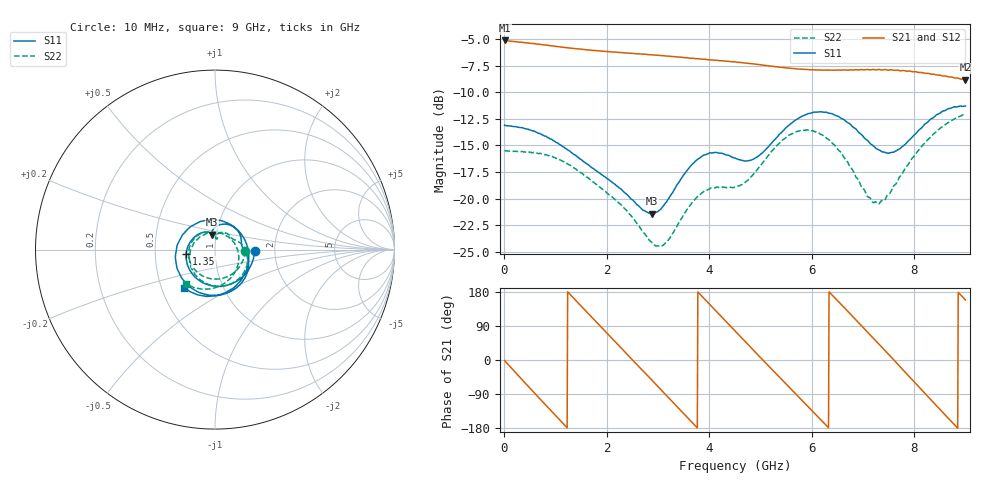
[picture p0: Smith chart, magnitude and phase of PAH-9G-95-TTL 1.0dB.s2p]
! MTS Systemtechnik GmbH
! S-Parameters
! Model: PAH-9G/95-TTL
! Attenuation Step: 1.0dB
#  HZ  S  DB  R  50.00
! Rohde & Schwarz Vector Network Analyzer
! Rohde-Schwarz,ZNB20-2Port,1334333062101652,3.45
! Created: UTC 1/26/2024, 7:17:38 AM
! freq[Hz]  db:S11  ang:S11  db:S21  ang:S21  db:S12  ang:S12  db:S22  ang:S22
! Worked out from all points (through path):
!   900 points, 10 MHz to 9 GHz, reference 50 ohm
!   highest |S21| = -5.13 dB at 10 MHz (marker M1); lowest = -8.8 dB at 9 GHz (marker M2)
!   group delay of S21, straight-line fit = 393 ps
!   lowest |S11| = -21.4 dB at 2.88 GHz (marker M3), VSWR 1.19, Z = 47.8 + j8.02 ohm
!   |S11| at or under -10 dB: start of sweep to end of sweep
!   |S22| runs from -24.5 to -12.1 dB; largest |S21 - S12| = 0.015
!   S11 on the Smith chart (normalised r, x): 10 MHz: 1.57, -0.03; 1.35 GHz: 0.72, -0.04; 9 GHz: 0.65, -0.30
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1e7  -13.10 -2.3  -5.13 -1.5  -5.13 -1.5  -15.47 -2.8
6.4e8  -13.78 -88.6  -5.47 -94.0  -5.47 -93.9  -15.72 -100.6
1.02e9  -14.73 -136.3  -5.69 -148.8  -5.70 -148.7  -16.23 -153.0
1.35e9  -15.81 -171.5  -5.88 164.1  -5.88 164.3  -17.07 169.0
1.51e9  -16.34 173.7  -5.96 141.3  -5.97 141.5  -17.59 152.8
1.91e9  -17.77 141.6  -6.13 84.7  -6.14 84.8  -19.10 120.1
2.32e9  -19.30 115.3  -6.28 26.6  -6.29 26.6  -20.80 94.1
2.88e9  -21.42 100.8  -6.48 -52.7  -6.48 -52.8  -24.11 78.3
3.01e9  -21.18 101.5  -6.53 -71.3  -6.53 -71.2  -24.47 81.2
3.34e9  -19.00 95.2  -6.65 -118.4  -6.66 -117.7  -22.88 86.9
3.76e9  -16.37 69.5  -6.84 -177.7  -6.85 -177.3  -19.88 70.0
4.17e9  -15.70 39.0  -7.00 124.3  -7.01 124.7  -18.93 46.5
4.51e9  -16.21 18.3  -7.15 76.2  -7.15 76.6  -18.90 33.0
5.14e9  -15.21 -6.6  -7.50 -13.1  -7.51 -12.1  -16.04 8.0
5.59e9  -12.97 -38.8  -7.75 -75.9  -7.76 -74.9  -13.98 -29.8
6.01e9  -11.93 -80.5  -7.88 -134.3  -7.90 -133.1  -13.61 -74.3
6.43e9  -12.10 -128.6  -7.92 167.3  -7.92 168.4  -14.90 -125.6
6.87e9  -13.48 173.1  -7.88 105.1  -7.90 106.5  -18.01 168.8
7.51e9  -15.72 63.7  -7.91 13.8  -7.88 14.7  -19.56 35.6
8.22e9  -12.96 -50.9  -8.21 -89.4  -8.21 -87.8  -14.72 -64.0
8.64e9  -11.62 -97.5  -8.51 -150.2  -8.56 -148.0  -12.92 -102.5
9e9  -11.30 -129.0  -8.83 158.4  -8.87 160.2  -12.07 -130.7
